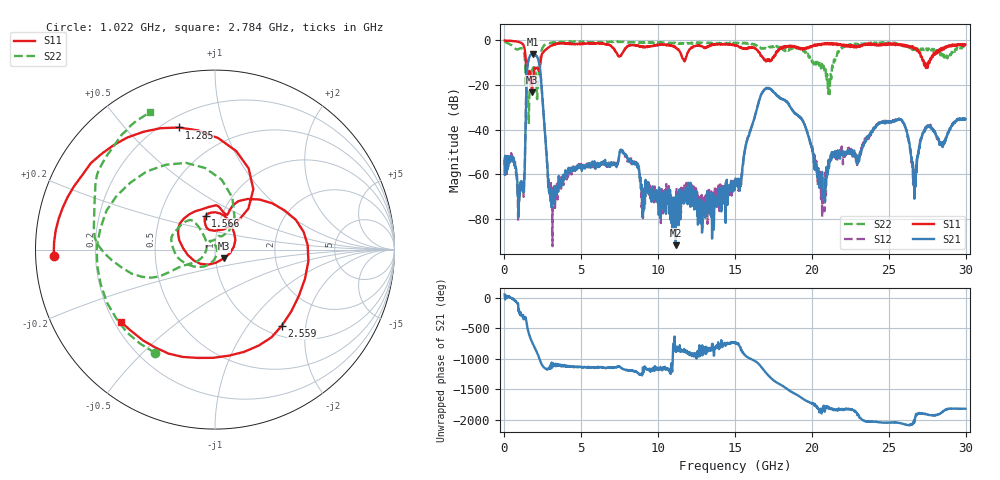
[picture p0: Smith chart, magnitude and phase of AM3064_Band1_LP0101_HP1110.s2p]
# Hz S DB R 50.0
!freq dBS11 angS11 dBS21 angS21 dBS12 angS12 dBS22 angS22
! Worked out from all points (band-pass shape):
!   1600 points, 10 MHz to 29.98 GHz, reference 50 ohm
!   highest |S21| = -6.05 dB at 1.828 GHz (marker M1); lowest = -91.8 dB at 11.14 GHz (marker M2)
!   |S21| within 3 dB of the highest: 1.552 GHz to 2.219 GHz (667.7 MHz wide, 35.4 % of centre)
!   lowest |S11| = -23.2 dB at 1.791 GHz (marker M3), VSWR 1.15, Z = 54.8 - j5.43 ohm
!   |S11| at or under -10 dB: 1.393 GHz to 2.343 GHz (950.3 MHz wide, 50.9 % of centre); 27.28222 GHz to 27.35566 GHz (73.44 MHz wide, 0.269 % of centre); 27.36 GHz to 27.57 GHz (211.5 MHz wide, 0.77 % of centre)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
!   |S22| runs from -37.5 to -0.4 dB; largest |S21 - S12| = 0.0083
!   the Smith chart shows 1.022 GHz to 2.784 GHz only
!   S11 on the Smith chart (normalised r, x): 1.022 GHz: 0.05, -0.02; 1.285 GHz: 0.26, +0.71; 1.566 GHz: 0.84, +0.33; 2.559 GHz: 1.18, -1.48; 2.784 GHz: 0.23, -0.33
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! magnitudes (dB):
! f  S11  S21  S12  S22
! 10 MHz  0.0  -53.0  -53.5  -0.4
! 1.022 GHz  -0.9  -66.9  -65.8  -3.5
! 1.285 GHz  -3.0  -64.3  -63.1  -5.9
! 1.566 GHz  -14.2  -8.6  -8.6  -33.0
! 1.791 GHz  -23.2  -6.1  -6.1  -13.3
! 1.828 GHz  -20.8  -6.1  -6.0  -12.7
! 2.559 GHz  -5.0  -34.1  -34.0  -2.3
! 2.784 GHz  -3.6  -55.6  -54.7  -1.4
! 3.159 GHz  -2.0  -73.2  -72.6  -1.0
! 5.015 GHz  -1.4  -56.3  -57.2  -0.7
! 7.657 GHz  -5.8  -49.4  -49.2  -0.7
! 10 GHz  -2.0  -71.0  -70.1  -0.9
! 11.14 GHz  -3.5  -91.8  -75.9  -1.4
! 15 GHz  -2.2  -65.2  -62.5  -1.4
! 17.03 GHz  -9.3  -21.2  -21.4  -3.7
! 19.99 GHz  -3.0  -47.9  -48.3  -9.2
! 20.76 GHz  -1.3  -69.4  -62.9  -11.3
! 25 GHz  -1.3  -36.6  -36.3  -1.2
! 25.99 GHz  -2.1  -37.4  -37.7  -2.2
! 26.66 GHz  -3.2  -70.9  -65.5  -4.0
! 27.43 GHz  -12.1  -38.7  -39.3  -3.9
! 29.98 GHz  -1.8  -35.3  -35.5  -2.8
